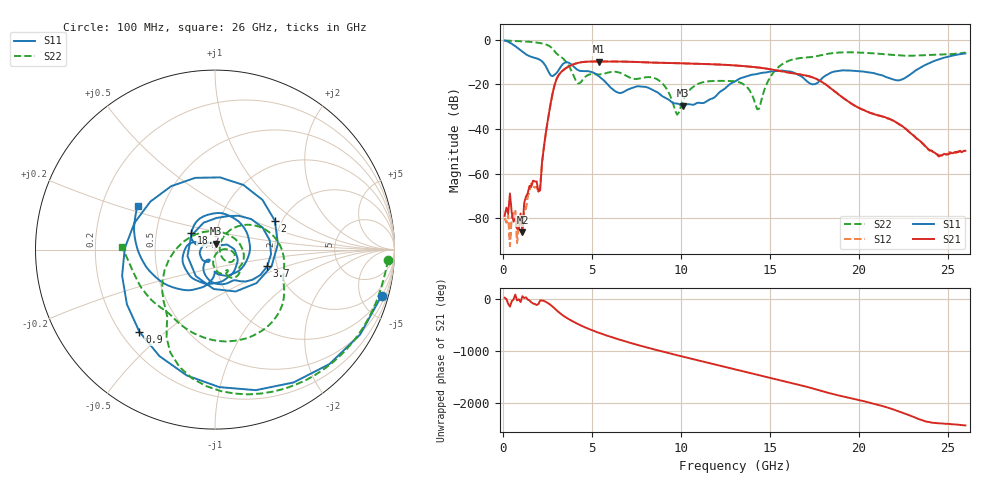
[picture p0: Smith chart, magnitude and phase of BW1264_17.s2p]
!Keysight Technologies,N5245B,MY57181159,A.13.60.06
!Date: Friday, December 18, 2020 23:52:49
!Correction: S11(Full 2 Port(1,2))
!S21(Full 2 Port(1,2))
!S12(Full 2 Port(1,2))
!S22(Full 2 Port(1,2))
!S2P File: Measurements: S11, S21, S12, S22:
# Hz S  dB  R 50
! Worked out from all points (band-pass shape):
!   260 points, 100 MHz to 26 GHz, reference 50 ohm
!   highest |S21| = -9.75 dB at 5.4 GHz (marker M1); lowest = -86.4 dB at 1.1 GHz (marker M2)
!   |S21| within 3 dB of the highest: 3.544 GHz to 14.66 GHz (11.12 GHz wide, 122 % of centre)
!   lowest |S11| = -29.6 dB at 10.1 GHz (marker M3), VSWR 1.07, Z = 50.4 + j3.32 ohm
!   |S11| at or under -10 dB: 2.239 GHz to 24.1 GHz (21.86 GHz wide, 166 % of centre)
!   |S22| runs from -33.6 to -0.3 dB; largest |S21 - S12| = 0.00052
!   S11 on the Smith chart (normalised r, x): 100 MHz: 1.02, -7.21; 900 MHz: 0.27, -0.41; 2 GHz: 1.83, +0.69; 3.7 GHz: 1.77, -0.36; 18.2 GHz: 0.76, +0.14; 26 GHz: 0.36, +0.23
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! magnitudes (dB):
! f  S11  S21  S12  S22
! 100 MHz  -0.3  -79.0  -80.0  -0.3
! 400 MHz  -1.3  -68.9  -92.6  -0.4
! 600 MHz  -2.3  -81.6  -77.7  -0.5
! 900 MHz  -4.1  -85.0  -83.8  -0.6
! 1.1 GHz  -5.4  -86.4  -85.4  -0.7
! 1.5 GHz  -7.3  -65.5  -67.9  -0.9
! 2 GHz  -8.6  -68.1  -68.4  -1.4
! 2.9 GHz  -15.8  -20.6  -20.6  -5.1
! 3.7 GHz  -10.3  -12.0  -12.0  -11.6
! 4.5 GHz  -14.0  -10.0  -10.0  -17.8
! 5.4 GHz  -16.4  -9.7  -9.7  -15.5
! 8.8 GHz  -24.2  -10.3  -10.3  -18.4
! 9.8 GHz  -28.6  -10.5  -10.5  -33.6
! 10.1 GHz  -29.6  -10.6  -10.6  -28.0
! 13.1 GHz  -18.5  -11.5  -11.5  -18.7
! 14.4 GHz  -15.1  -12.5  -12.5  -31.0
! 15.4 GHz  -14.0  -13.7  -13.7  -12.9
! 17.4 GHz  -20.0  -16.8  -16.8  -7.7
! 18.2 GHz  -15.8  -20.3  -20.3  -6.4
! 21.7 GHz  -17.1  -35.4  -35.4  -6.6
! 24.5 GHz  -8.8  -52.3  -51.6  -6.7
! 26 GHz  -6.1  -49.8  -49.9  -5.7
